PROGRAM PRG_FileFindEnumList
VAR
	fbEnum			: FB_EnumFindFileList := ( sNetID := '', tTimeout := T#5S, sPathName := 'D:\temp\*.*', pFindList := ADR(filesList), cbFindList := SIZEOF(filesList));
	filesList 		: ARRAY[1..10] OF ST_FindFileEntry;
	bFirst			: BOOL;
	bNext			: BOOL;
	bAbort			: BOOL;
	bBusy			: BOOL;
	bError			: BOOL;
	nErrID			: UDINT;
	bEOE			: BOOL;
	nFindFiles		: UDINT;
	nState 			: BYTE;
END_VAR

CASE nState OF
	0:
		IF bFirst XOR  bNext XOR bAbort THEN 
			fbEnum( bExecute := FALSE );
			fbEnum( bExecute := TRUE,  eCmd := SEL(bAbort, SEL(bFirst, eEnumCmd_Next, eEnumCmd_First), eEnumCmd_Abort));
			bFirst := bNext := bAbort := FALSE;
			nState	:= 1;
		END_IF

	1:	(* wait until function block not busy *)
		fbEnum( bExecute := FALSE );
		IF NOT fbEnum.bBusy THEN
			IF NOT fbEnum.bError THEN
				IF NOT fbEnum.bEOE THEN
					ADSLOGSTR( ADSLOG_MSGTYPE_HINT OR ADSLOG_MSGTYPE_LOG, 'FB_EnumFindFileList.nFindFiles=%s', UDINT_TO_STRING(fbEnum.nFindFiles));
					//bNext := TRUE; 
					nState 	:= 0;
				ELSE (* no more entries *)
					nState 	:= 0;
				END_IF
			ELSE (* log error *)
				ADSLOGSTR( ADSLOG_MSGTYPE_ERROR OR ADSLOG_MSGTYPE_LOG, 'FB_EnumFindFileList.Error=%s', DWORD_TO_HEXSTR( fbEnum.nErrID, 0, FALSE ) );
				nState 	:= 0;
			END_IF
		END_IF
END_CASE

END_PROGRAM
